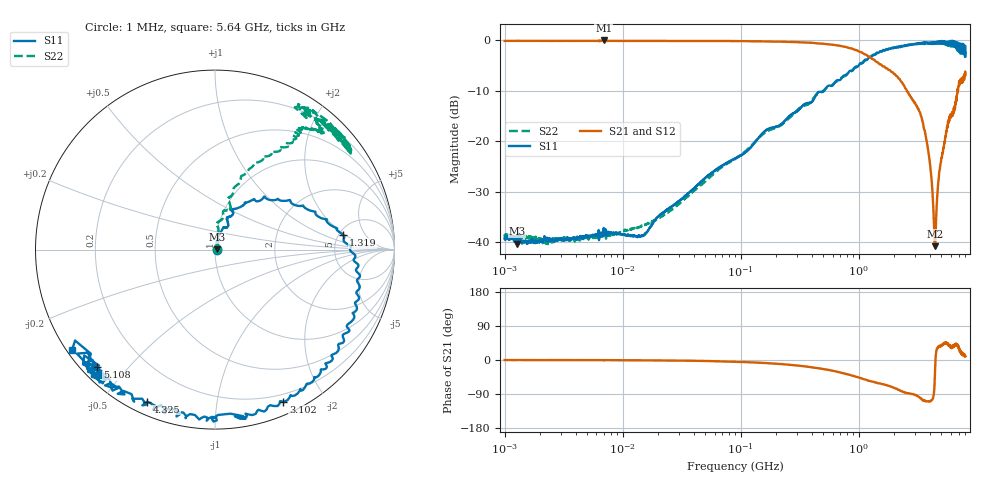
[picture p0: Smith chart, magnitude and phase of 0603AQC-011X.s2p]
!s-Parameter Generated by FASTRON Sdn. Bhd.
!FASTRON P/N : 0603AQC-011X
!Keysight Technologies: E5071C_MY46733604_B.14.02
!Date: Thu Jun 25 13:51:34 2026
!Version  :Rev00  Thu Jun 25 13:51:34 2026
!Data & Calibration Information:
!Freq  S11:SOLT2(ON)  S21:SOLT2(ON)  S12:SOLT2(ON)  S22:SOLT2(ON)
!PortZ  Port1:50+j0  Port2:50+j0
!When reading reference impedance value at option line is always used.
! Remarks : This data is being provided solely for informational purposes.
# Hz S dB R 50
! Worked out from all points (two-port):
!   1601 points, 1 MHz to 8 GHz, reference 50 ohm
!   highest |S21| = -0.01 dB at 6.912 MHz (marker M1); lowest = -40.8 dB at 4.409 GHz (marker M2)
!   |S21| within 3 dB of the highest: start of sweep to 1.18 GHz
!   lowest |S11| = -40.3 dB at 1.271 MHz (marker M3), VSWR 1.02, Z = 51 + j0.115 ohm
!   |S11| at or under -10 dB: start of sweep to 507.9 MHz
!   |S22| runs from -40.4 to -0.4 dB; largest |S21 - S12| = 0.012
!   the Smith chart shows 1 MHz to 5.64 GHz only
!   S11 on the Smith chart (normalised r, x): 1 MHz: 1.02, -0.00; 1.319 GHz: 5.44, +1.84; 3.102 GHz: 0.12, -1.54; 4.325 GHz: 0.05, -0.65; 5.108 GHz: 0.04, -0.41; 5.64 GHz: 0.02, -0.32
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1000000  -39.30 -1.5  -0.10 -0.1  -0.10 -0.1  -38.90 4.2
1270633  -40.30 6.7  -0.11 -0.1  -0.10 -0.1  -39.20 -2.4
4479405  -38.80 15.8  -0.11 -0.3  -0.11 -0.3  -39.30 18.4
6911657  -37.20 12.6  -0.01 -0.8  -0.05 -0.4  -37.60 19.2
1.46648e7  -38.80 33.3  -0.10 -0.8  -0.11 -0.8  -36.80 39.4
2.00676e7  -34.90 42.7  -0.11 -1.1  -0.11 -1.0  -35.30 55.8
8.994653e7  -23.40 76.9  -0.14 -4.6  -0.15 -4.6  -23.50 72.3
4.006501e8  -12.20 66.2  -0.47 -19.4  -0.47 -19.4  -11.90 70.0
8.33667e8  -6.11 33.8  -1.53 -39.0  -1.52 -39.1  -6.25 67.1
1.318613e9  -2.88 6.6  -3.75 -57.2  -3.75 -57.4  -2.96 55.8
1.7949e9  -1.68 -13.5  -5.87 -68.1  -5.90 -68.3  -1.66 54.2
2.296158e9  -1.09 -35.4  -8.22 -81.7  -8.25 -81.8  -1.17 49.9
3.102129e9  -0.63 -65.8  -13.00 -94.4  -13.00 -94.3  -0.71 52.6
3.791269e9  -0.45 -92.5  -20.50 -109.0  -20.50 -109.0  -0.53 44.9
4.054764e9  -0.46 -103.0  -25.60 -109.0  -25.60 -109.0  -0.57 46.1
4.324643e9  -0.66 -114.0  -35.70 -89.5  -35.70 -89.8  -0.73 47.5
4.408619e9  -0.68 -116.0  -40.80 -43.7  -40.90 -44.1  -0.74 46.7
5.108415e9  -0.66 -135.0  -22.30 39.7  -22.30 39.4  -0.61 43.9
5.64026e9  -0.26 -145.0  -17.30 42.5  -17.20 42.3  -0.70 56.3
6.110812e9  -0.45 -162.0  -14.80 31.0  -14.80 30.8  -0.96 45.7
6.65058e9  -0.72 -152.0  -12.20 43.5  -12.10 43.1  -0.97 75.0
8e9  -1.23 151.0  -6.88 9.4  -6.92 8.8  -2.24 65.3
